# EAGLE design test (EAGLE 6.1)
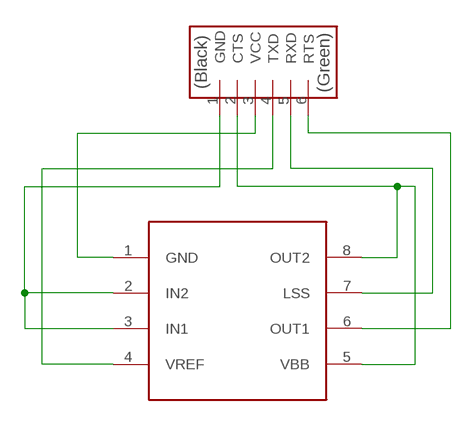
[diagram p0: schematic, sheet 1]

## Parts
U$1  A4953  A4953-H-BRIDGE-MOTOR-DRIVER  [SOIC8]
U$2  FTDI-SMD-HEADER  [1X06SMD]

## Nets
N$1: U$1.1(GND) U$2.3(VCC)
N$2: U$1.2(IN2) U$1.3(IN1) U$2.1(GND)
N$4: U$1.4(VREF) U$2.4(TXD)
N$6: U$1.7(LSS) U$2.5(RXD)
N$7: U$1.6(OUT1) U$2.6(RTS)
N$8: U$1.5(VBB) U$1.8(OUT2) U$2.2(CTS)

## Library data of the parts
U$1 = fab:A4953-H-BRIDGE-MOTOR-DRIVER
U$2 = fab:FTDI-SMD-HEADER

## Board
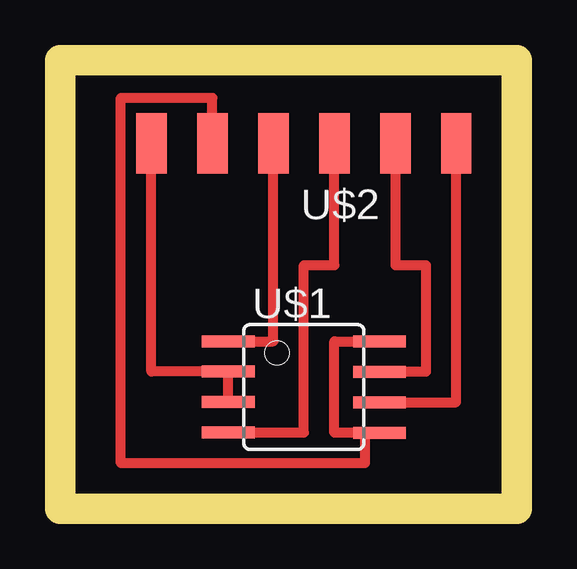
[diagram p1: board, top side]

Size 19.03 x 18.72 mm. Coordinates in mm from the lower left corner, seen from the top.
Outline: 0,0 19.03,0 19.03,18.72 0,18.72 0,0
Copper layers (1*16): Top 0.035mm / dielectric 1.5mm / Bottom 0.035mm
Design rules: minimum track width 10mil, minimum drill 24mil, track to track 8mil, track to pad 8mil, pad to pad 8mil, via to via 8mil, smd to smd 8mil, copper to edge 40mil, drill to drill 8mil, minimum pad ring 10mil, minimum via ring 8mil, stop-mask expansion 4mil, vias tented up to drill 0mil, thermal gap 10mil

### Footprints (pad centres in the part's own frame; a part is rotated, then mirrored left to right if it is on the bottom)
SOIC8 = smd 0.5 x 2.2: 1 -1.905,-3.154; 2 -0.645,-3.154; 3 0.625,-3.154; 4 1.895,-3.154; 5 1.905,3.154; 6 0.635,3.154; 7 -0.635,3.154; 8 -1.905,3.154
1X06SMD = smd 2.54 x 1.27: 1 0,6.35; 2 0,3.81; 3 0,1.27; 4 0,-1.27; 5 0,-3.81; 6 0,-6.35

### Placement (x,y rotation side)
U$1  10.16,5.08 270 top
U$2  10.16,15.24 90 top

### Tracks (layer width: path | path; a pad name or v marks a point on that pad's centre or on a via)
N$1
  Top 0.406: U$1.1 8.89,6.99 U$2.3
N$2
  Top 0.406: U$1.3 U$1.2 3.81,5.72 U$2.1
N$4
  Top 0.406: U$1.4 10.16,3.19 10.16,10.16 11.43,10.16 U$2.4
N$6
  Top 0.406: U$2.5 13.97,10.16 15.24,10.16 15.24,5.71 U$1.7
N$7
  Top 0.406: U$1.6 16.51,4.45 U$2.6
N$8
  Top 0.406: U$2.2 6.35,17.14 2.54,17.14 2.54,1.91 12.7,1.91 12.7,3.17 U$1.5 11.43,3.17 11.43,6.99 U$1.8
